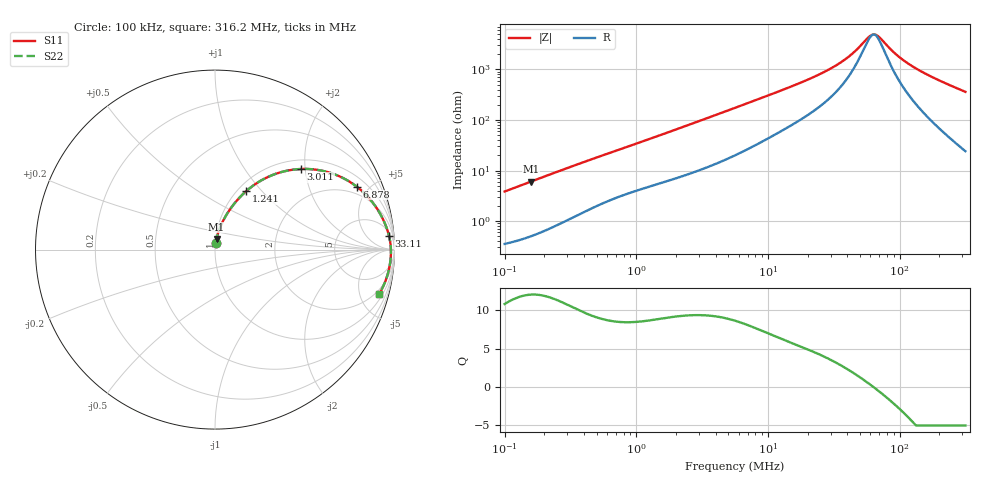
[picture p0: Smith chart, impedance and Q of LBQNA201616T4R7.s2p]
! LBQNA201616T4R7  S-PARAMETER MODEL  ( General Type )
! Model Generated by TAIYO YUDEN Corporation (http://www.ty-top.com)
! Version 1.0
! TAIYO YUDEN Control No. 191025NI43SB-FBB
! Copyright(c) 2019 TAIYO YUDEN CO.,LTD. All Rights Reserved.
! Product Description (link to TY-COMPAS)
! https://ds.yuden.co.jp/TYCOMPAS/or/detail?pn=LBQNA201616T4R7M&u=M
! Products Name : Inductors
! Characteristics :
!  Inductance : 4.7 uH , SRF(min) : 45 MHz , DC Resistance(max) : 0.325 Ohm
!  Rated Current : Saturation :340 mA , Temp Rise : 410 mA (20 degC)
!  Case Size : 2.0 x 1.6 / 0.079 x 0.063 [mm/inch] , Thickness : 1.6 / 0.063 [mm/inch]
!  (Conditions: Temperature = 25 degC , DC Bias Current/Voltage = 0A / 0V)
! External Node Assignments :
!  1  o---GGG---o  2
! GND o---------o GND
! Frequency Range : 0.1MHz  -  316.199832MHz  [ 402 STEP ]
# MHz S RI R 50
! Freq[MHz].  S11 Real  S11 Imag  S21 Real  S21 Imag  S12 Real  S12 Imag  S22 Real  S22 Imag
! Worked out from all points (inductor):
!   401 points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, 100 kHz to 316.2 MHz, reference 50 ohm
!   read as one part in series: L = 6.06 uH near 104.1 kHz
!   highest Q = 12.1 at 158.9 kHz (marker M1), where L = 6.04 uH
!   self-resonance near 63.49 MHz
!   S11 on the Smith chart (normalised r, x): 100 kHz: 1.01, +0.08; 1.241 MHz: 1.09, +0.82; 3.011 MHz: 1.20, +1.90; 6.878 MHz: 1.51, +4.20; 33.11 MHz: 8, +23; 316.2 MHz: 1.48, -7.21
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0.1  0.00495 0.0379  0.995 -0.0379  0.995 -0.0379  0.00495 0.0379
0.158945  0.00855 0.0595  0.9914 -0.0595  0.9914 -0.0595  0.00855 0.0595
0.385695  0.033 0.1349  0.967 -0.1349  0.967 -0.1349  0.033 0.1349
0.734921  0.0854 0.2269  0.9146 -0.2269  0.9146 -0.2269  0.0854 0.2269
1.240904  0.1734 0.3253  0.8266 -0.3253  0.8266 -0.3253  0.1734 0.3253
1.487603  0.219 0.3611  0.781 -0.3611  0.781 -0.3611  0.219 0.3611
3.01116  0.4789 0.4491  0.5211 -0.4491  0.5211 -0.4491  0.4789 0.4491
4.073637  0.6076 0.437  0.3924 -0.437  0.3924 -0.437  0.6076 0.437
5.623165  0.7288 0.3906  0.2712 -0.3906  0.2712 -0.3906  0.7288 0.3906
6.87828  0.7899 0.3507  0.2101 -0.3507  0.2101 -0.3507  0.7899 0.3507
11.38223  0.8919 0.244  0.1081 -0.244  0.1081 -0.244  0.8919 0.244
21.68824  0.9523 0.1316  0.0477 -0.1316  0.0477 -0.1316  0.9523 0.1316
33.11101  0.9701 0.0744  0.0299 -0.0744  0.0299 -0.0744  0.9701 0.0744
43.02502  0.9761 0.0433  0.0239 -0.0433  0.0239 -0.0433  0.9761 0.0433
57.04529  0.9795 0.0118  0.0205 -0.0118  0.0205 -0.0118  0.9795 0.0118
61.83287  0.98 0.00291  0.02 -0.00291  0.02 -0.00291  0.98 0.00291
68.38627  0.9803 -0.0082  0.0197 0.0082  0.0197 0.0082  0.9803 -0.0082
83.65039  0.98 -0.0309  0.02 0.0309  0.02 0.0309  0.98 -0.0309
104.4039  0.978 -0.0573  0.022 0.0573  0.022 0.0573  0.978 -0.0573
138.4253  0.9724 -0.0949  0.0276 0.0949  0.0276 0.0949  0.9724 -0.0949
202.9849  0.9563 -0.1565  0.0437 0.1565  0.0437 0.1565  0.9563 -0.1565
316.1998  0.9145 -0.2481  0.0855 0.2481  0.0855 0.2481  0.9145 -0.2481
